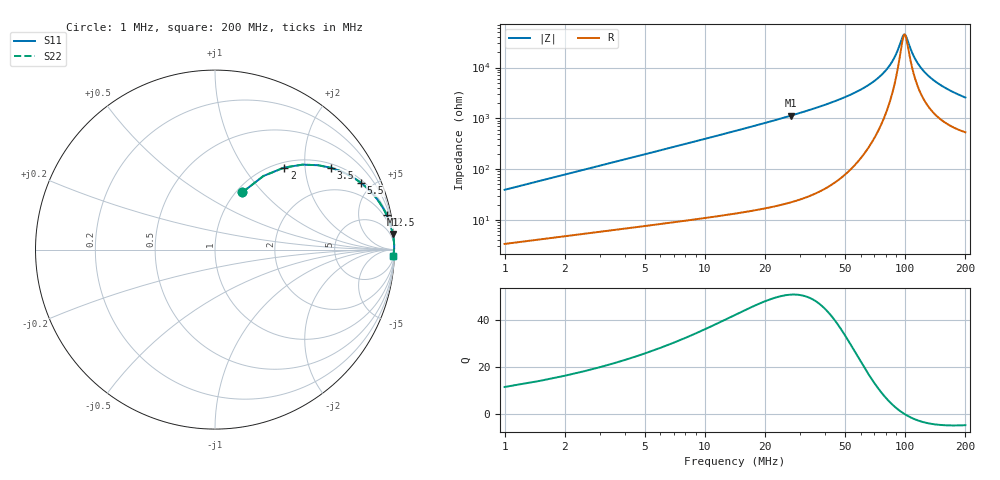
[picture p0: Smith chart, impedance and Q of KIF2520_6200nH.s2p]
!version-2
!date-12.2020
!Series
# MHz S RI R 50
!Freq ReS11 ImS11 ReS21 ImS21 ReS12 ImS12 ReS22 ImS22
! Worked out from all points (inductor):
!   399 points, 1 MHz to 200 MHz, reference 50 ohm
!   read as one part in series: L = 6.2 uH near 1.5 MHz
!   highest Q = 51 at 27 MHz (marker M1), where L = 6.7 uH
!   self-resonance near 99.5 MHz
!   S11 on the Smith chart (normalised r, x): 1 MHz: 1.07, +0.78; 2 MHz: 1.10, +1.56; 3.5 MHz: 1.13, +2.73; 5.5 MHz: 1.16, +4.30; 12.5 MHz: 1.25, +9.90; 200 MHz: 12, -50
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1  0.1529 0.3193  0.8471 -0.3193  0.8471 -0.3193  0.1529 0.3193
1.5  0.2697 0.41  0.7303 -0.41  0.7303 -0.41  0.2697 0.41
2  0.3855 0.4572  0.6145 -0.4572  0.6145 -0.4572  0.3855 0.4572
3.5  0.6449 0.456  0.3551 -0.456  0.3551 -0.456  0.6449 0.456
5.5  0.8134 0.3716  0.1866 -0.3716  0.1866 -0.3716  0.8134 0.3716
8  0.9007 0.2841  0.0993 -0.2841  0.0993 -0.2841  0.9007 0.2841
12.5  0.9564 0.1922  0.0436 -0.1922  0.0436 -0.1922  0.9564 0.1922
19  0.9808 0.1272  0.0192 -0.1272  0.0192 -0.1272  0.9808 0.1272
27  0.9906 0.087  0.00937 -0.087  0.00937 -0.087  0.9906 0.087
34.5  0.9944 0.0649  0.00557 -0.0649  0.00557 -0.0649  0.9944 0.0649
67.5  0.9983 0.0204  0.00174 -0.0204  0.00174 -0.0204  0.9983 0.0204
83.5  0.9982 0.00903  0.00178 -0.00903  0.00178 -0.00903  0.9982 0.00903
90  0.9981 0.00515  0.00193 -0.00515  0.00193 -0.00515  0.9981 0.00515
97.5  0.9978 0.00105  0.00215 -0.00105  0.00215 -0.00105  0.9978 0.00105
99  0.9978 0.000266  0.00221 -0.000266  0.00221 -0.000266  0.9978 0.000266
100.5  0.9977 -0.000502  0.00226 0.000502  0.00226 0.000502  0.9977 -0.000502
108  0.9974 -0.00417  0.00257 0.00417  0.00257 0.00417  0.9974 -0.00417
114  0.9971 -0.00694  0.00285 0.00694  0.00285 0.00694  0.9971 -0.00694
122.5  0.9967 -0.0106  0.0033 0.0106  0.0033 0.0106  0.9967 -0.0106
134  0.996 -0.0153  0.00399 0.0153  0.00399 0.0153  0.996 -0.0153
167  0.9936 -0.0271  0.0064 0.0271  0.0064 0.0271  0.9936 -0.0271
200  0.9906 -0.0374  0.00939 0.0374  0.00939 0.0374  0.9906 -0.0374
